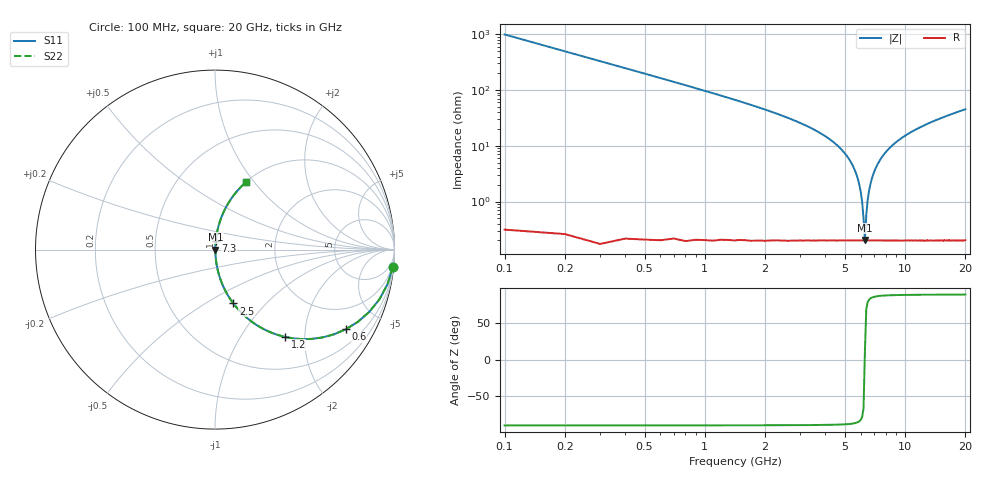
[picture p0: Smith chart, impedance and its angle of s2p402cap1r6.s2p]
! AVX Thin Film Operation		Date: April 2003
! Description: Accu-P® Series, Thin Film, SMD, RF Capacitor
! Part Number: 04021J1R6ABS
! 50 MHz  -  20 GHz
! Serial Measurements
# hz S db R 50
!	S11		S21		S12		S22
!	dB	Phase	dB	Phase	dB	Phase	dB	Phase
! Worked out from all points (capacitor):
!   200 points, 100 MHz to 20 GHz, reference 50 ohm
!   read as one part in series: C = 1.6 pF near 200 MHz
!   lowest |Z| = 205 mohm at 6.3 GHz (marker M1)
!   series resonance near 6.291 GHz, so ESL is about 400 pH
!   S11 on the Smith chart (normalised r, x): 100 MHz: 1, -20; 600 MHz: 1.00, -3.29; 1.2 GHz: 1.00, -1.60; 2.5 GHz: 1.00, -0.67; 7.3 GHz: 1.00, +0.09; 20 GHz: 1.00, +0.91
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1e8  -0.04 -5.7  -20.00 84.2  -20.00 84.2  -0.04 -5.7
2e8  -0.17 -11.4  -14.10 78.6  -14.10 78.6  -0.17 -11.4
3e8  -0.38 -16.8  -10.77 73.2  -10.77 73.2  -0.38 -16.8
6e8  -1.37 -31.3  -5.68 58.6  -5.68 58.6  -1.37 -31.3
1.2e9  -4.11 -51.3  -2.15 38.6  -2.15 38.6  -4.11 -51.3
1.8e9  -6.90 -62.9  -1.01 26.9  -1.01 26.9  -6.90 -62.9
2.5e9  -9.97 -71.2  -0.48 18.5  -0.48 18.5  -9.97 -71.2
3.5e9  -14.32 -78.3  -0.18 11.1  -0.18 11.1  -14.32 -78.3
4.8e9  -21.30 -83.7  -0.05 4.9  -0.05 4.9  -21.30 -83.7
5.6e9  -28.67 -84.8  -0.02 2.1  -0.02 2.1  -28.67 -84.8
6e9  -36.43 -81.5  -0.02 0.9  -0.02 0.9  -36.43 -81.5
6.1e9  -40.05 -77.9  -0.02 0.6  -0.02 0.6  -40.05 -77.9
6.3e9  -53.79 12.5  -0.02 -0.0  -0.02 -0.0  -53.79 12.5
6.4e9  -44.78 69.5  -0.02 -0.3  -0.02 -0.3  -44.78 69.5
6.5e9  -39.58 78.5  -0.02 -0.6  -0.02 -0.6  -39.58 78.5
6.8e9  -32.17 84.0  -0.02 -1.4  -0.02 -1.4  -32.17 84.0
7.3e9  -26.54 84.9  -0.03 -2.7  -0.03 -2.7  -26.54 84.9
8.4e9  -20.71 83.5  -0.05 -5.3  -0.05 -5.3  -20.71 83.5
1.01e10  -16.29 80.5  -0.12 -8.8  -0.12 -8.8  -16.29 80.5
1.34e10  -11.92 74.9  -0.31 -14.7  -0.31 -14.7  -11.92 74.9
1.67e10  -9.41 69.9  -0.55 -19.8  -0.55 -19.8  -9.41 69.9
2e10  -7.70 65.4  -0.82 -24.3  -0.82 -24.3  -7.70 65.4
